PROGRAM MAIN
VAR
	TestStart		:BOOL := 1;	
	
	//config parameter
	ModuleNum 		:BYTE := 4;
	TestPosNum		:BYTE := 2;
	TestPosStart	:BYTE := 0;
	Pos				:ARRAY[0..9] OF DINT :=[20000,0,0,0,0,0,0,0,0,0];
	Spd				:ARRAY[0..9] OF INT  :=[100,300,0,0,0,0,0,0,0,0];
	
	
	TestState 		:UINT := 0;
	ModuleIndex		:BYTE := 0;
	
	CommandWord				AT %Q* : ARRAY[0..15] OF UINT;
	TargetPos				AT %Q* : ARRAY[0..15] OF DINT;
	TargetSpd				AT %Q* : ARRAY[0..15] OF INT;
	
	
	FeedbackWord   			AT %I* : ARRAY[0..15] OF UINT;
	ActualPos				AT %I* : ARRAY[0..15] OF DINT;
	ActualSpd				AT %I* : ARRAY[0..15] OF INT;
	
	
	
	TestCnt		 	:UINT := 0;
	
END_VAR


IF (TestStart = 1) THEN 
	

	CASE TestState OF
		
		0: 
			FOR ModuleIndex:= 0 TO (ModuleNum-1) BY 1 DO
				CommandWord[ModuleIndex] := 17;
				TargetPos[ModuleIndex] := Pos[TestPosStart];
				TargetSpd[ModuleIndex] := Spd[TestPosStart];
			END_FOR
			
			TestPosStart := TestPosStart+1;
			IF(TestPosStart = TestPosNum)THEN
				TestPosStart := 0;
			END_IF
			
			TestState := 1;
			
		1: 
			TestCnt := 0;
			
			FOR ModuleIndex:= 0 TO (ModuleNum-1) BY 1 DO
				
				IF (FeedbackWord[ModuleIndex] = 1) THEN
					TestCnt := TestCnt+1;
				END_IF
			
			END_FOR
			
			IF (TestCnt = ModuleNum)THEN
				TestState := 2;
			END_IF
		
		2:
			TestCnt := 0;
			
			FOR ModuleIndex:= 0 TO (ModuleNum-1) BY 1 DO
				
				IF (FeedbackWord[ModuleIndex] = 3) THEN
					TestCnt := TestCnt+1;
				END_IF
			
			END_FOR
			
			IF (TestCnt = ModuleNum)THEN
				TestState := 3;
			END_IF
			
		3..250:
			TestState := TestState+1;
			
		251:
			TestState := 0;

	     ELSE
		    TestState := TestState;
		
	END_CASE

	
	
ELSE
	
	FOR ModuleIndex:= 0 TO (ModuleNum-1) BY 1 DO
		CommandWord[ModuleIndex] := 0;
		TargetPos[ModuleIndex] := 0;
		TargetSpd[ModuleIndex] := 0;
	END_FOR
			
	TestState := 0;
	
END_IF

END_PROGRAM
